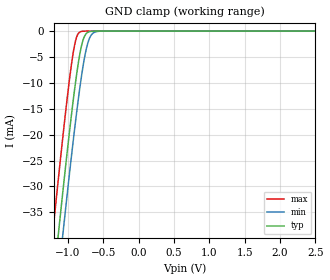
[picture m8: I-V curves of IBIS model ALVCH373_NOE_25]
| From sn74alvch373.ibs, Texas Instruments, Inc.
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[Model]   ALVCH373_NOE_25
Model_type  Input
Vinl=0.7
Vinh=1.7
| variable   typ   min   max
C_comp   3.64pF   3.11pF   4.38pF
[Temperature Range]   40   100   -40
| Ambient temperature   25   85   -40
[Voltage range]   2.5   2.3   2.7
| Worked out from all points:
|   GND clamp passes 1 mA (typ) near -0.77 V on its own axis
[GND Clamp]
| ALVCH373_NOE_25
|   Voltage   I(typ)   I(min)   I(max)
-2.5V     -228.1mA   -235.8mA   -218.5mA
-1.23V    -51.59mA   -59.87mA   -40.97mA
-1.2V     -47.61mA   -55.9mA    -36.97mA
-1.13V    -38.42mA   -46.71mA   -27.77mA
-1.07V    -30.71mA   -38.96mA   -20.13mA
-925mV    -13.29mA   -21.11mA   -4.122mA
-880mV    -8.606mA   -15.99mA   -1.263mA
-830mV    -4.281mA   -10.75mA   -171.6uA
-780mV    -1.472mA   -6.227mA   -17.15uA
-720mV    -242.5uA   -2.354mA   -1.023uA
-600mV    -3.832uA   -109.2uA   -3.608nA
2.5V      4.713pA    7.577pA    4.389pA
